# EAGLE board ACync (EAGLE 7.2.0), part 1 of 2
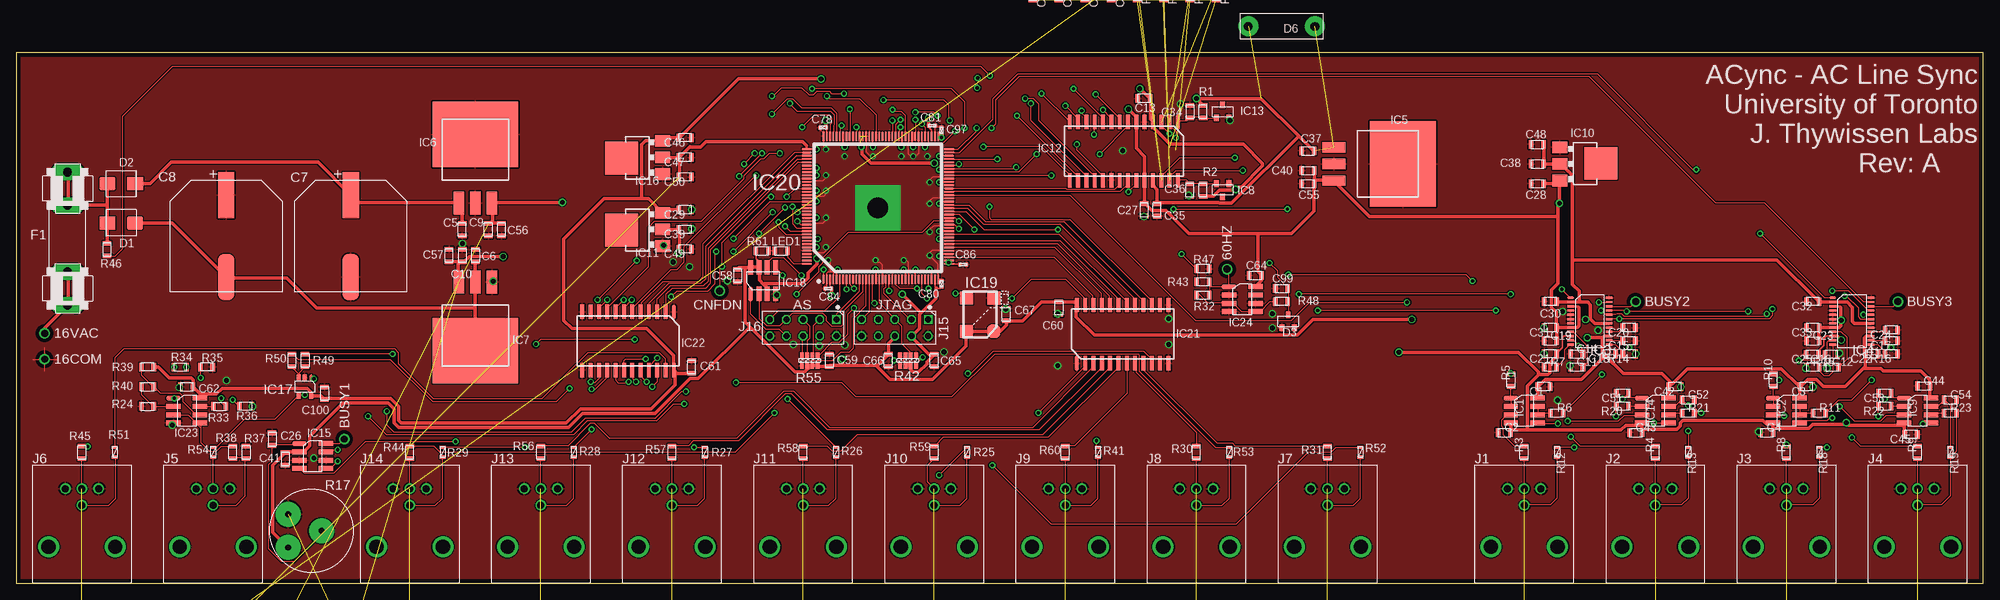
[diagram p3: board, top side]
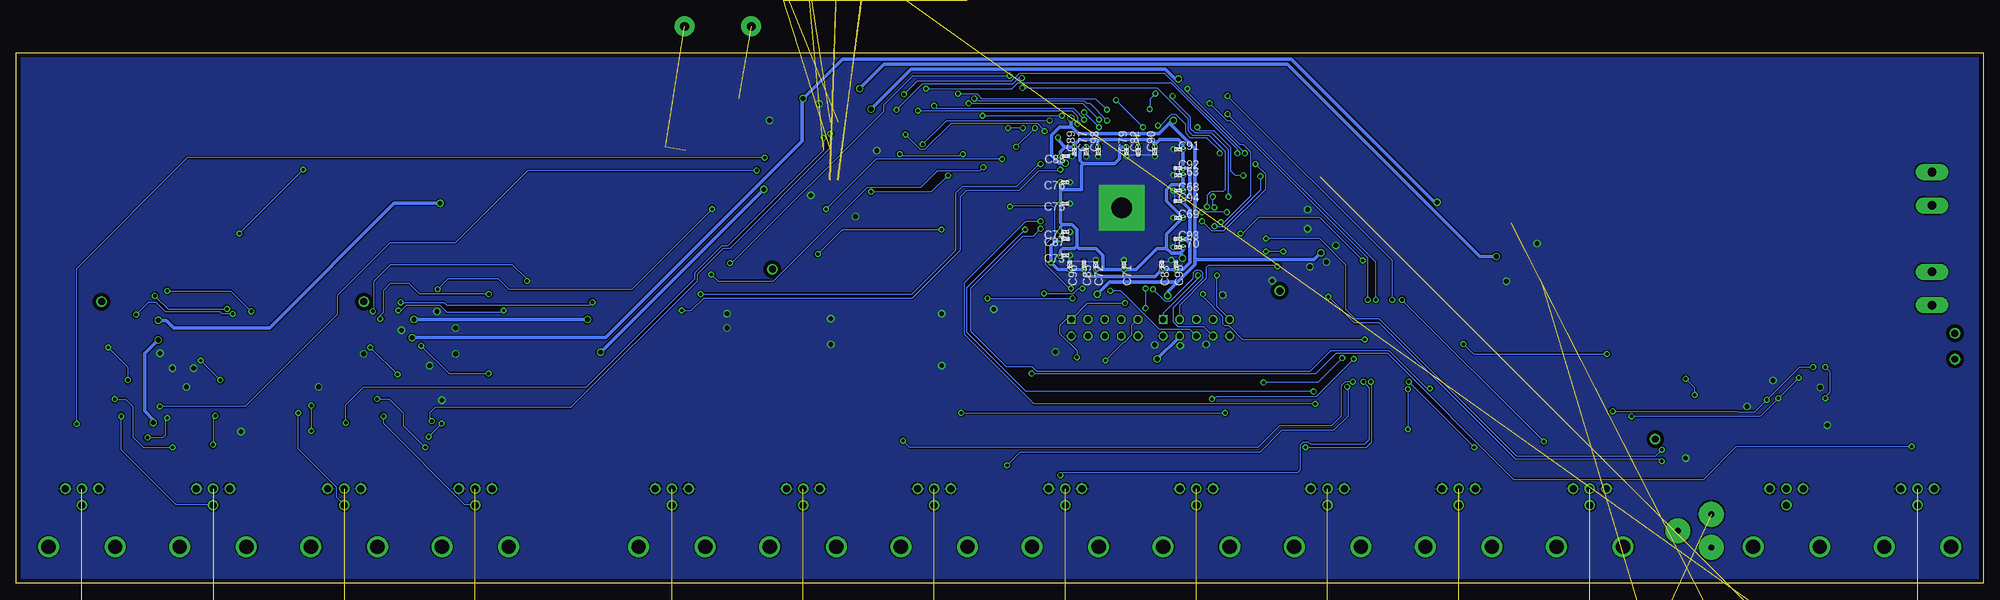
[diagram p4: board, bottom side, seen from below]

Size 300 x 81 mm. Coordinates in mm from the lower left corner, seen from the top.
Outline: 0,0 300,0 300,81 0,81 0,0
Copper layers (1+16): Top 0.035mm / dielectric 1.5mm / Bottom 0.035mm
Design rules "DRC standard check": minimum track width 0.18mm, minimum drill 20mil, track to track 0.18mm, track to pad 0.18mm, pad to pad 0.18mm, via to via 0.18mm, smd to smd 0mil, copper to edge 25mil, drill to drill 0.18mm, minimum pad ring 0.18mm, minimum via ring 0.203mm, stop-mask expansion 4mil, vias tented up to drill 0mil, thermal gap 10mil
Net classes: 0 default: width 0.18 mm, drill 0.508 mm, clearance 0.18 mm; 1 Power: width 0.25 mm, drill 0.711 mm, clearance 0.18 mm; 2 Power-isolated: width 0.5 mm, drill 0.711 mm, clearance 0.5 mm

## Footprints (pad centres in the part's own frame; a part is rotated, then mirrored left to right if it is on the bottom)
TP-0.042B = drill 1.067: TP 0,0
2012(0805) = smd 0.7 x 1.3: 1 -0.95,0; 2 0.95,0
CAP,POL,16MM,PLASTIC_BASE = smd 7 x 2.5: NEG -6.26,0; POS 6.25,0
1005(0402) = smd 0.5 x 0.6: 1 -0.5,0; 2 0.5,0
EIA-B(SMB) = smd 2.4 x 2: A- -2.11,0; K+ 2.11,0
SOT23 = smd 0.75 x 1: 1 -0.95,-1; 2 0.95,-1; 3 0,1
PASSIVE_0.4" = drill 1.321 pad 3.048: 1 -5.08,0; 2 5.08,0
FUSE = drill 1.321 pad 2.54 long: 1A -10.16,0; 1B -5.08,0; 2A 10.16,0; 2B 5.08,0
SOIC-8 = smd 0.75 x 2.2: 1 -1.27,-2.032; 2 0,-2.032; 3 1.27,-2.032; 4 2.54,-2.032; 5 2.54,2.032; 6 1.27,2.032; 7 0,2.032; 8 -1.27,2.032
TSSOP-24 = smd 0.356 x 1.016: 1 -3.575,-2.925; 2 -2.925,-2.925; 3 -2.275,-2.925; 4 -1.625,-2.925; 5 -0.975,-2.925; 6 -0.325,-2.925; 7 0.325,-2.925; 8 0.975,-2.925; 9 1.625,-2.925; 10 2.275,-2.925; 11 2.925,-2.925; 12 3.575,-2.925; 13 3.575,2.925; 14 2.925,2.925; 15 2.275,2.925; 16 1.625,2.925; 17 0.975,2.925; 18 0.325,2.925; 19 -0.325,2.925; 20 -0.975,2.925; 21 -1.625,2.925; 22 -2.275,2.925; 23 -2.925,2.925; 24 -3.575,2.925
D2PAK = smd 1.6 x 3.5: 1 -2.54,0; 2 0,0; 3 2.54,0 | smd 13 x 10: TAB 0,10.5
SOT223 = smd 1.778 x 2.3: 1 -2.54,-2.54; 3 2.54,-2.54 | smd 1.778 x 2.286: 2 0,-2.54 | smd 5 x 5: 4 -0.1,3.7
SOIC28 = smd 0.6 x 2.2: 1 -8.255,-4.445; 2 -6.985,-4.445; 3 -5.715,-4.445; 4 -4.445,-4.445; 5 -3.175,-4.445; 6 -1.905,-4.445; 7 -0.635,-4.445; 8 0.635,-4.445; 9 1.905,-4.445; 10 3.175,-4.445; 11 4.445,-4.445; 12 5.715,-4.445; 13 6.985,-4.445; 14 8.255,-4.445; 15 8.255,4.445; 16 6.985,4.445; 17 5.715,4.445; 18 4.445,4.445; 19 3.175,4.445; 20 1.905,4.445; 21 0.635,4.445; 22 -0.635,4.445; 23 -1.905,4.445; 24 -3.175,4.445; 25 -4.445,4.445; 26 -5.715,4.445; 27 -6.985,4.445; 28 -8.255,4.445
SOT23-5 = smd 0.6 x 1: 1 -0.95,-1.35; 2 0,-1.35; 3 0.95,-1.35; 4 0.95,1.35; 5 -0.95,1.35
CSX750(CITIZEN_OSC) = smd 2 x 2: 1 -2.54,-2.1; 2 2.54,-2.1; 3 2.54,2.1; 4 -2.54,2.1
EQFP144(TQFP_WITH_GROUND_PAD) = smd 1.5 x 0.27: 1 -10.89,8.29; 2 -10.89,7.79; 3 -10.89,7.29; 4 -10.89,6.79; 5 -10.89,6.29; 6 -10.89,5.79; 7 -10.89,5.29; 8 -10.89,4.79; 9 -10.89,4.29; 10 -10.89,3.79; 11 -10.89,3.29; 12 -10.89,2.79; 13 -10.89,2.29; 14 -10.89,1.79; 15 -10.89,1.29; 16 -10.89,0.79; 17 -10.89,0.29; 18 -10.89,-0.21; 19 -10.89,-0.71; 20 -10.89,-1.21; 21 -10.89,-1.71; 22 -10.89,-2.21; 23 -10.89,-2.71; 24 -10.89,-3.21; 25 -10.89,-3.71; 26 -10.89,-4.21; 27 -10.89,-4.71; 28 -10.89,-5.21; 29 -10.89,-5.71; 30 -10.89,-6.21; 31 -10.89,-6.71; 32 -10.89,-7.21; 33 -10.89,-7.71; 34 -10.89,-8.21; 35 -10.89,-8.71; 36 -10.89,-9.21; 73 10.91,-9.21; 74 10.91,-8.71; 75 10.91,-8.21; 76 10.91,-7.71; 77 10.91,-7.21; 78 10.91,-6.71; 79 10.91,-6.21; 80 10.91,-5.71; 81 10.91,-5.21; 82 10.91,-4.71; 83 10.91,-4.21; 84 10.91,-3.71; 85 10.91,-3.21; 86 10.91,-2.71; 87 10.91,-2.21; 88 10.91,-1.71; 89 10.91,-1.21; 90 10.91,-0.71; 91 10.91,-0.21; 92 10.91,0.29; 93 10.91,0.79; 94 10.91,1.29; 95 10.91,1.79; 96 10.91,2.29; 97 10.91,2.79; 98 10.91,3.29; 99 10.91,3.79; 100 10.91,4.29; 101 10.91,4.79; 102 10.91,5.29; 103 10.91,5.79; 104 10.91,6.29; 105 10.91,6.79; 106 10.91,7.29; 107 10.91,7.79; 108 10.91,8.29 | smd 0.27 x 1.5: 37 -8.54,-10.86; 38 -8.04,-10.86; 39 -7.54,-10.86; 40 -7.04,-10.86; 41 -6.54,-10.86; 42 -6.04,-10.86; 43 -5.54,-10.86; 44 -5.04,-10.86; 45 -4.54,-10.86; 46 -4.04,-10.86; 47 -3.54,-10.86; 48 -3.04,-10.86; 49 -2.54,-10.86; 50 -2.04,-10.86; 51 -1.54,-10.86; 52 -1.04,-10.86; 53 -0.54,-10.86; 54 -0.04,-10.86; 55 0.46,-10.86; 56 0.96,-10.86; 57 1.46,-10.86; 58 1.96,-10.86; 59 2.46,-10.86; 60 2.96,-10.86; 61 3.46,-10.86; 62 3.96,-10.86; 63 4.46,-10.86; 64 4.96,-10.86; 65 5.46,-10.86; 66 5.96,-10.86; 67 6.46,-10.86; 68 6.96,-10.86; 69 7.46,-10.86; 70 7.96,-10.86; 71 8.46,-10.86; 72 8.96,-10.86; 109 8.96,10.84; 110 8.46,10.84; 111 7.96,10.84; 112 7.46,10.84; 113 6.96,10.84; 114 6.46,10.84; 115 5.96,10.84; 116 5.46,10.84; 117 4.96,10.84; 118 4.46,10.84; 119 3.96,10.84; 120 3.46,10.84; 121 2.96,10.84; 122 2.46,10.84; 123 1.96,10.84; 124 1.46,10.84; 125 0.96,10.84; 126 0.46,10.84; 127 -0.04,10.84; 128 -0.54,10.84; 129 -1.04,10.84; 130 -1.54,10.84; 131 -2.04,10.84; 132 -2.54,10.84; 133 -3.04,10.84; 134 -3.54,10.84; 135 -4.04,10.84; 136 -4.54,10.84; 137 -5.04,10.84; 138 -5.54,10.84; 139 -6.04,10.84; 140 -6.54,10.84; 141 -7.04,10.84; 142 -7.54,10.84; 143 -8.04,10.84; 144 -8.54,10.84 | drill 3.175 pad 7 square: PAD 0,0
SOIC24 = smd 0.6 x 2.2: 1 -6.985,-4.445; 2 -5.715,-4.445; 3 -4.445,-4.445; 4 -3.175,-4.445; 5 -1.905,-4.445; 6 -0.635,-4.445; 7 0.635,-4.445; 8 1.905,-4.445; 9 3.175,-4.445; 10 4.445,-4.445; 11 5.715,-4.445; 12 6.985,-4.445; 13 6.985,4.445; 14 5.715,4.445; 15 4.445,4.445; 16 3.175,4.445; 17 1.905,4.445; 18 0.635,4.445; 19 -0.635,4.445; 20 -1.905,4.445; 21 -3.175,4.445; 22 -4.445,4.445; 23 -5.715,4.445; 24 -6.985,4.445
CONN:BNC,DUAL(BOMAR) = drill 1.067: LWR-COM 14.45,-2.54; LWR-CTR 11.91,0; UPR-COM 14.45,2.54; UPR-CTR 14.45,0 | drill 2.184: MTG1 5.56,-5.08; MTG2 5.56,5.08
CONN,2X5,BLASTER,UNSHROUDED = drill 0.889 square: 1 -1.27,5.08 | drill 0.889 octagon: 2 1.27,5.08; 3 -1.27,2.54; 4 1.27,2.54; 5 -1.27,0; 6 1.27,0; 7 -1.27,-2.54; 8 1.27,-2.54; 9 -1.27,-5.08; 10 1.27,-5.08
1608(0603) = smd 0.5 x 0.9: 1 -0.75,0; 2 0.75,0
PRECISION-SPR-RV8(POT) = drill 0.889 pad 3.81: CCW -2.54,-3.531; CW 2.54,-3.531; W 0,1.549
PANASONIC_EXB-V8V(QUAD-R-PACK) = smd 0.9 x 0.59: 1A -0.8,1.2; 1B 0.8,1.2; 2A -0.8,0.4; 2B 0.8,0.4; 3A -0.8,-0.4; 3B 0.8,-0.4; 4A -0.8,-1.2; 4B 0.8,-1.2

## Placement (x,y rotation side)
16COM  5002  [TP-0.042B]  4.32,34.2 0 top
16VAC  5002  [TP-0.042B]  4.32,38.16 0 top
60HZ  [TP-0.042B]  184.68,47.96 90 top
AC  WAU16-400  [MISC]  not placed on the board
BUSY1  [TP-0.042B]  50,22 270 top
BUSY2  [TP-0.042B]  247,43 0 top
BUSY3  [TP-0.042B]  287,43 0 top
C1  0.1uF  [2012(0805)]  233,30 180 top
C2  0.1uF  [2012(0805)]  227,23 0 top
C3  0.1uF  [2012(0805)]  273,30 180 top
C4  0.1uF  [2012(0805)]  267,23 0 top
C5  0.1uF  [2012(0805)]  68,54 90 top
C6  0.1uF  [2012(0805)]  70,50 270 top
C7  1000uF  [CAP,POL,16MM,PLASTIC_BASE]  51,53 90 top
C8  1000uF  [CAP,POL,16MM,PLASTIC_BASE]  32,53 90 top
C9  0.1uF  [2012(0805)]  72,54 90 top
C10  0.1uF  [2012(0805)]  68,50 270 top
C11  0.1uF  [2012(0805)]  238,33 0 top
C12  0.1uF  [2012(0805)]  277,33 0 top
C13  0.1uF  [2012(0805)]  172,74 180 top
C14  1nF  [2012(0805)]  238,35 0 top
C15  1nF  [2012(0805)]  246,37 180 top
C16  1nF  [2012(0805)]  276.84,34.92 180 top
C17  1nF  [2012(0805)]  286,37 180 top
C18  0.1uF  [2012(0805)]  243,35 180 top
C19  10uF  [2012(0805)]  234,37 0 top
C20  0.1uF  [2012(0805)]  246,39 180 top
C21  0.1uF  [2012(0805)]  234,35 180 top
C22  0.1uF  [2012(0805)]  283,35 180 top
C23  10uF  [2012(0805)]  274,37 0 top
C24  0.1uF  [2012(0805)]  286,38.64 180 top
C25  0.1uF  [2012(0805)]  273.96,34.92 180 top
C26  0.1uF  [2012(0805)]  39,22 270 top
C27  0.1uF  [2012(0805)]  172,57 270 top
C28  0.1uF  [2012(0805)]  232,61 0 top
C29  0.1uF  [2012(0805)]  102,57 180 top
C30  0.1uF  [2012(0805)]  234,43 180 top
C31  0.1uF  [2012(0805)]  234,39 180 top
C32  0.1uF  [2012(0805)]  274,43 180 top
C33  0.1uF  [2012(0805)]  274,39 180 top
C34  0.1uF  [2012(0805)]  179,72 270 top
C35  0.1uF  [2012(0805)]  174,57 90 top
C36  0.1uF  [2012(0805)]  179,60 90 top
C37  0.1uF  [2012(0805)]  197,66 0 top
C38  0.1uF  [2012(0805)]  232,64 0 top
C39  0.1uF  [2012(0805)]  102,54 180 top
C40  0.1uF  [2012(0805)]  197,63 0 top
C41  0.1uF  [2012(0805)]  41,19 270 top
C42  0.1uF  [2012(0805)]  253,30 180 top
C43  0.1uF  [2012(0805)]  247,23 0 top
C44  0.1uF  [2012(0805)]  290.92,30.12 0 top
C45  0.1uF  [2012(0805)]  289,22.72 180 top
C46  0.1uF  [2012(0805)]  102,68 180 top
C47  0.1uF  [2012(0805)]  102,65 180 top
C48  10uF  [2012(0805)]  232,67 0 top
C49  10uF  [2012(0805)]  102,51 180 top
C50  10uF  [2012(0805)]  102,62 180 top
C51  0.1uF  [2012(0805)]  245,29 180 top
C52  0.1uF  [2012(0805)]  255,28 0 top
C53  0.1uF  [2012(0805)]  285,29 180 top
C54  0.1uF  [2012(0805)]  295,28 0 top
C55  10uF  [2012(0805)]  197,61 0 top
C56  10uF  [2012(0805)]  74,54 90 top
C57  10uF  [2012(0805)]  66,50 90 top
C58  0.1uF  [2012(0805)]  110,47 270 top
C59  0.1uF  [2012(0805)]  124,34 270 top
C60  0.1uF  [2012(0805)]  159,42 270 top
C61  0.1uF  [2012(0805)]  103,33 90 top
C62  0.1uF  [2012(0805)]  26,30 0 top
C63  0.1uF  [1005(0402)]  122.76,62.28 0 bottom
C64  0.1uF  [2012(0805)]  189,47 0 top
C65  0.1uF  [2012(0805)]  140,34 90 top
C66  0.1uF  [2012(0805)]  133,34 90 top
C67  0.1uF  [2012(0805)]  151,41 90 top
C68  0.1uF  [1005(0402)]  122.76,59.94 0 bottom
C69  0.1uF  [1005(0402)]  122.76,55.8 0 bottom
C70  0.1uF  [1005(0402)]  122.76,51.3 0 bottom
C71  0.1uF  [1005(0402)]  131.04,48.6 270 bottom
C72  0.1uF  [1005(0402)]  135.36,48.6 270 bottom
C73  0.1uF  [1005(0402)]  140.04,50.04 180 bottom
C74  0.1uF  [1005(0402)]  140.04,53.64 180 bottom
C75  0.1uF  [1005(0402)]  140.04,57.96 180 bottom
C76  0.1uF  [1005(0402)]  140.04,61.2 180 bottom
C77  0.1uF  [1005(0402)]  136.8,65.88 90 bottom
C78  0.1uF  [1005(0402)]  123.08,69.56 0 top
C79  0.1uF  [1005(0402)]  130.68,65.88 90 bottom
C80  0.1uF  [1005(0402)]  141.12,45.72 270 top
C81  0.1uF  [1005(0402)]  139.68,69.84 180 top
C82  0.1uF  [1005(0402)]  128.88,65.88 90 bottom
C83  0.1uF  [1005(0402)]  125.28,48.6 270 bottom
C84  0.1uF  [1005(0402)]  123.84,45 0 top
C85  0.1uF  [1005(0402)]  137.16,48.6 270 bottom
C86  0.1uF  [1005(0402)]  144.44,48.64 180 top
C87  0.1uF  [1005(0402)]  140.04,52.56 180 bottom
C88  0.1uF  [1005(0402)]  139.96,65.2 180 bottom
C89  0.1uF  [1005(0402)]  138.6,65.88 90 bottom
C90  0.1uF  [1005(0402)]  126.36,65.88 90 bottom
C91  0.1uF  [1005(0402)]  122.76,66.24 0 bottom
C92  0.1uF  [1005(0402)]  122.76,63.36 0 bottom
C93  0.1uF  [1005(0402)]  122.76,52.56 0 bottom
C94  0.1uF  [1005(0402)]  122.76,58.32 0 bottom
C95  0.1uF  [1005(0402)]  123.12,48.6 270 bottom
C96  0.1uF  [1005(0402)]  139.32,48.6 270 bottom
C97  0.1uF  [1005(0402)]  141.12,69.12 270 top
C98  0.1uF  [1005(0402)]  135,65.88 90 bottom
C99  0.1uF  [2012(0805)]  193,45 0 top
C100  0.1uF  [2012(0805)]  47,29 270 top
C101  1nF  [2012(0805)]  not placed on the board
C102  1nF  [2012(0805)]  not placed on the board
C103  1nF  [2012(0805)]  not placed on the board
C104  1nF  [2012(0805)]  not placed on the board
CASE1  PBPA19001UNF  [MISC]  not placed on the board
CASE2  Custom cover  [MISC]  not placed on the board
CNFDN  [TP-0.042B]  107.28,44.64 180 top
D1  STTH4R02U  [EIA-B(SMB)]  16,55 180 top
D2  STTH4R02U  [EIA-B(SMB)]  16,61 0 top
D3  BAS70-04  [SOT23]  194,40 0 top
D4  STTH4R02U  [EIA-B(SMB)]  not placed on the board
D5  STTH4R02U  [EIA-B(SMB)]  not placed on the board
D6  1N5339  [PASSIVE_0.4"]  not placed on the board
F1  0.4A  [FUSE]  7.81,52.6 90 top
IC1  ADA4001-2AR  [SOIC-8]  230,27 270 top
IC2  ADA4001-2AR  [SOIC-8]  270,27 270 top
IC3  AD7366BRU  [TSSOP-24]  240,40 270 top
IC4  AD7366BRU  [TSSOP-24]  280,40 270 top
IC5  L7805CDT  [D2PAK]  201,64 270 top
IC6  L7815ACD2T  [D2PAK]  70,58 0 top
IC7  MC7915ACD2T  [D2PAK]  70,46 180 top
IC8  LM4040DIM3-10.0  [SOT23]  184,60 180 top
IC9  ADA4001-2AR  [SOIC-8]  290,27 270 top
IC10  LM1117MPX-3.3  [SOT223]  238,64 270 top
IC11  LM1117MPX-2.5  [SOT223]  96,54 90 top
IC12  DAC7724U  [SOIC28]  168.93,65.97 180 top
IC13  LM4040DIM3-10.0  [SOT23]  184,72 0 top
IC14  ADA4001-2AR  [SOIC-8]  250,27 270 top
IC15  AD7896JR  [SOIC-8]  45.19,20.06 270 top
IC16  LM1117MPX-ADJ  [SOT223]  96,65 90 top
IC17  AD8605ART  [SOT23-5]  44,30 180 top
IC18  EPCS4  [SOIC-8]  113.26,46.19 0 top
IC19  ASV-100.000MHZ-E-C-T  [CSX750(CITIZEN_OSC)]  147,41 90 top
IC20  EP4CE15E22C6  [EQFP144(TQFP_WITH_GROUND_PAD)]  131.4,57.3 90 top
IC21  SN74LVC827ADW  [SOIC24]  168.75,38.03 0 top
IC22  SN74ABT2827DWR  [SOIC24]  93.3,36.97 180 top
IC23  TLV3202AIDR  [SOIC-8]  26,27 270 top
IC24  TLV3202AIDR  [SOIC-8]  187,44 270 top
J1  364A  [CONN:BNC,DUAL(BOMAR)]  230,0 90 top
J2  364A  [CONN:BNC,DUAL(BOMAR)]  250,0 90 top
J3  364A  [CONN:BNC,DUAL(BOMAR)]  270,0 90 top
J4  364A  [CONN:BNC,DUAL(BOMAR)]  290,0 90 top
J5  364A2595  [CONN:BNC,DUAL(BOMAR)]  30,0 90 top
J6  364A2595  [CONN:BNC,DUAL(BOMAR)]  10,0 90 top
J7  364A2595  [CONN:BNC,DUAL(BOMAR)]  200,0 90 top
J8  364A2595  [CONN:BNC,DUAL(BOMAR)]  180,0 90 top
J9  364A2595  [CONN:BNC,DUAL(BOMAR)]  160,0 90 top
J10  364A2595  [CONN:BNC,DUAL(BOMAR)]  140,0 90 top
J11  364A2595  [CONN:BNC,DUAL(BOMAR)]  120,0 90 top
J12  364A2595  [CONN:BNC,DUAL(BOMAR)]  100,0 90 top
J13  364A2595  [CONN:BNC,DUAL(BOMAR)]  80,0 90 top
J14  364A2595  [CONN:BNC,DUAL(BOMAR)]  60,0 90 top
J15  XG4C-1031  [CONN,2X5,BLASTER,UNSHROUDED]  134,39 270 top
J16  XG4C-1031  [CONN,2X5,BLASTER,UNSHROUDED]  120,39 270 top
KNOB  8567  [MISC]  not placed on the board
LED1  SML-211YTT86  [2012(0805)]  116.64,50.76 0 top
NUT1  364KNT  [MISC]  not placed on the board
NUT2  364KNT  [MISC]  not placed on the board
NUT3  364KNT  [MISC]  not placed on the board
NUT4  364KNT  [MISC]  not placed on the board
NUT5  364KNT  [MISC]  not placed on the board
NUT6  364KNT  [MISC]  not placed on the board
NUT7  364KNT  [MISC]  not placed on the board
NUT8  364KNT  [MISC]  not placed on the board
NUT9  364KNT  [MISC]  not placed on the board
NUT10  364KNT  [MISC]  not placed on the board
NUT11  364KNT  [MISC]  not placed on the board
NUT12  364KNT  [MISC]  not placed on the board
NUT13  364KNT  [MISC]  not placed on the board
NUT14  364KNT  [MISC]  not placed on the board
NUT15  364KNT  [MISC]  not placed on the board
NUT16  364KNT  [MISC]  not placed on the board
NUT17  364KNT  [MISC]  not placed on the board
NUT18  364KNT  [MISC]  not placed on the board
NUT19  364KNT  [MISC]  not placed on the board
NUT20  364KNT  [MISC]  not placed on the board
NUT21  364KNT  [MISC]  not placed on the board
NUT22  364KNT  [MISC]  not placed on the board
NUT23  364KNT  [MISC]  not placed on the board
NUT24  364KNT  [MISC]  not placed on the board
NUT25  364KNT  [MISC]  not placed on the board
NUT26  364KNT  [MISC]  not placed on the board
NUT27  364KNT  [MISC]  not placed on the board
NUT28  364KNT  [MISC]  not placed on the board
R1  1K  [2012(0805)]  181,72 90 top
R2  1K  [2012(0805)]  181,60 90 top
R3  100  [2012(0805)]  230,20 90 top
R4  100  [2012(0805)]  250,20 90 top
R5  100  [2012(0805)]  228,31 90 top
R6  100  [2012(0805)]  235,26 0 top
R7  100  [2012(0805)]  234,33 0 top
R8  100  [2012(0805)]  270,20 90 top
R9  100  [2012(0805)]  290,20 90 top
R10  100  [2012(0805)]  268,31 90 top
R11  100  [2012(0805)]  275,26 0 top
R12  47 (PTC)  [1608(0603)]  235,20 270 top
R13  47 (PTC)  [1608(0603)]  255,20 270 top
R14  100  [2012(0805)]  246,35 180 top
R15  100  [2012(0805)]  274,33 0 top
R16  100  [2012(0805)]  286,35 180 top
R17  SPRU1031S28  [PRECISION-SPR-RV8(POT)]  45,8 270 top
R18  47 (PTC)  [1608(0603)]  275,20 270 top
R19  47 (PTC)  [1608(0603)]  295,20 270 top
R20  1K  [2012(0805)]  245,27 180 top
R21  1K  [2012(0805)]  255,26 0 top
R22  1K  [2012(0805)]  285,27 180 top
R23  1K  [2012(0805)]  295,26 0 top
R24  4.99K  [2012(0805)]  20,27 0 top
R25  47(PTC)  [1608(0603)]  145,20 270 top
R26  47(PTC)  [1608(0603)]  125,20 270 top
R27  47(PTC)  [1608(0603)]  105,20 270 top
R28  47(PTC)  [1608(0603)]  85,20 270 top
R29  47(PTC)  [1608(0603)]  65,20 270 top
R30  100  [2012(0805)]  180,20 90 top
R31  100  [2012(0805)]  200,20 90 top
R32  1.2M  [2012(0805)]  181,44 0 top
R33  4.99K  [2012(0805)]  31,27 0 top
R34  4.99K  [2012(0805)]  25,33 0 top
R35  4.99K  [2012(0805)]  29,33 180 top
R36  4.99K  [2012(0805)]  35,27 180 top
R37  100K  [2012(0805)]  35,20 270 top
R38  4.99K  [2012(0805)]  33,20 90 top
R39  12.7K  [2012(0805)]  20,33 180 top
R40  4.99K  [2012(0805)]  20,30 0 top
R41  47(PTC)  [1608(0603)]  165,20 270 top
R42  1K  [PANASONIC_EXB-V8V(QUAD-R-PACK)]  136,34 90 top
R43  4.99K  [2012(0805)]  181,46 180 top
R44  100  [2012(0805)]  60,20 90 top
R45  100  [2012(0805)]  10,20 90 top
R46  10K  [2012(0805)]  13.8,50.92 270 top
R47  4.99K  [2012(0805)]  181,48 180 top
R48  4.99K  [2012(0805)]  193,43 180 top
R49  4.99K  [2012(0805)]  44,34 270 top
R50  4.99K  [2012(0805)]  42,34 270 top
R51  47(PTC)  [1608(0603)]  15,20 270 top
R52  47(PTC)  [1608(0603)]  205,20 270 top
R53  47(PTC)  [1608(0603)]  185,20 270 top
R54  47(PTC)  [1608(0603)]  30,20 270 top
R55  10K  [PANASONIC_EXB-V8V(QUAD-R-PACK)]  121,34 270 top
R56  100  [2012(0805)]  80,20 90 top
R57  100  [2012(0805)]  100,20 90 top
R58  100  [2012(0805)]  120,20 90 top
R59  100  [2012(0805)]  140,20 90 top
R60  100  [2012(0805)]  160,20 90 top
R61  365  [2012(0805)]  113.76,50.76 0 top
R62  365  [2012(0805)]  not placed on the board
R63  100K  [2012(0805)]  not placed on the board
R64  100K  [2012(0805)]  not placed on the board
R65  100K  [2012(0805)]  not placed on the board
R66  100K  [2012(0805)]  not placed on the board
R67  100K  [2012(0805)]  not placed on the board
R68  100K  [2012(0805)]  not placed on the board
R69  100K  [2012(0805)]  not placed on the board
R70  100K  [2012(0805)]  not placed on the board
R71  100K  [2012(0805)]  not placed on the board
R72  100K  [2012(0805)]  not placed on the board
R73  100K  [2012(0805)]  not placed on the board
R74  100K  [2012(0805)]  not placed on the board
R75  100K  [2012(0805)]  not placed on the board
R76  1.65K  [2012(0805)]  not placed on the board
R77  1.65K  [2012(0805)]  not placed on the board
R78  1.65K  [2012(0805)]  not placed on the board
R79  1.65K  [2012(0805)]  not placed on the board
